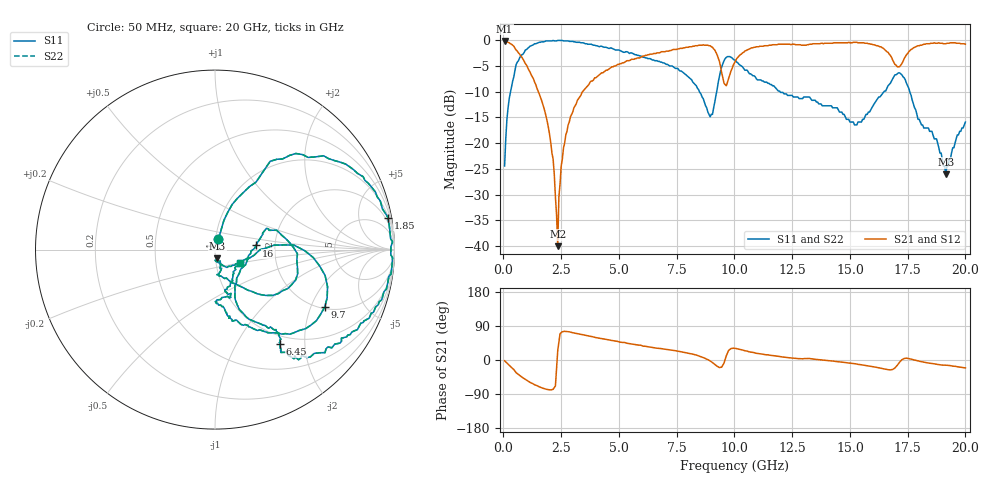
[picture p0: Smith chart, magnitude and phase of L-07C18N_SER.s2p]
#	mhz	s	ma	r	50
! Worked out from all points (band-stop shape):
!   400 points, 50 MHz to 20 GHz, reference 50 ohm
!   highest |S21| = -0.18 dB at 50 MHz (marker M1); lowest = -40.0 dB at 2.35 GHz (marker M2)
!   |S21| within 3 dB of the highest: 6.019 GHz to 9.276 GHz (3.257 GHz wide, 42.6 % of centre); 10.18 GHz to 16.78 GHz (6.592 GHz wide, 48.9 % of centre)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
!   lowest |S11| = -26.0 dB at 19.15 GHz (marker M3), VSWR 1.11, Z = 51.1 - j4.94 ohm
!   |S11| at or under -10 dB: 8.484 GHz to 9.234 GHz (749.4 MHz wide, 8.46 % of centre); 11.97 GHz to 16.48 GHz (4.513 GHz wide, 31.7 % of centre); 17.59 GHz to end of sweep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
!   |S22| runs from -26.0 to -0.1 dB; largest |S21 - S12| = 0
!   S11 on the Smith chart (normalised r, x): 50 MHz: 1.03, +0.12; 1.85 GHz: 1, +11; 6.45 GHz: 0.86, -1.54; 9.7 GHz: 2.08, -2.53; 16 GHz: 1.59, +0.08; 20 GHz: 1.31, -0.20
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50  0.06 72.3  0.98 -2.0  0.98 -2.0  0.06 72.3
200  0.22 71.1  0.95 -11.0  0.95 -11.0  0.22 71.1
550  0.58 58.0  0.8 -33.5  0.8 -33.5  0.58 58.0
1850  0.98 10.5  0.18 -77.1  0.18 -77.1  0.98 10.5
2150  0.99 2.5  0.07 -77.4  0.07 -77.4  0.99 2.5
2350  0.99 -2.6  0.01 24.6  0.01 24.6  0.99 -2.6
2400  0.99 -4.1  0.03 47.0  0.03 47.0  0.99 -4.1
2600  0.98 -8.8  0.09 75.2  0.09 75.2  0.98 -8.8
3400  0.94 -23.1  0.31 67.0  0.31 67.0  0.94 -23.1
6450  0.64 -55.6  0.73 33.1  0.73 33.1  0.64 -55.6
6700  0.62 -54.2  0.75 30.9  0.75 30.9  0.62 -54.2
8950  0.18 -36.8  0.88 -2.5  0.88 -2.5  0.18 -36.8
9350  0.44 3.3  0.62 -19.9  0.62 -19.9  0.44 3.3
9700  0.69 -27.5  0.39 18.4  0.39 18.4  0.69 -27.5
10050  0.63 -48.4  0.63 30.6  0.63 30.6  0.63 -48.4
11150  0.41 -76.4  0.87 15.9  0.87 15.9  0.41 -76.4
13350  0.26 -69.9  0.91 3.1  0.91 3.1  0.26 -69.9
16000  0.23 5.7  0.9 -17.6  0.9 -17.6  0.23 5.7
16700  0.37 14.8  0.73 -25.8  0.73 -25.8  0.37 14.8
17450  0.38 -42.2  0.72 4.8  0.72 4.8  0.38 -42.2
19150  0.05 -74.4  0.92 -13.7  0.92 -13.7  0.05 -74.4
20000  0.16 -27.6  0.91 -20.7  0.91 -20.7  0.16 -27.6
